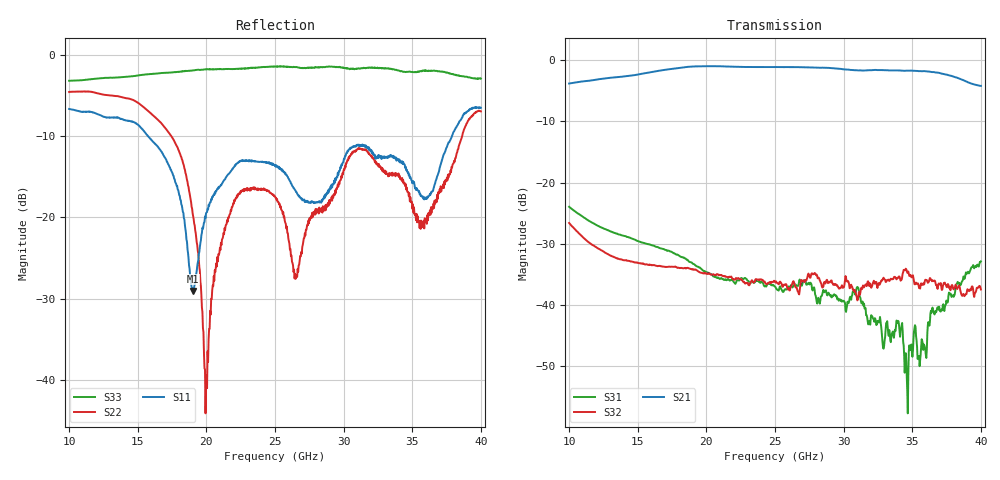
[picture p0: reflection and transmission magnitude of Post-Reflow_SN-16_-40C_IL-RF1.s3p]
!Agilent Technologies,N5245A,US49150155,A.09.90.19
!Agilent N5245A: A.09.90.19
!Date: Wednesday, November 14, 2018 00:00:33
!Correction: S11(Full 3 Port(1,2,3))
!S12(Full 3 Port(1,2,3))
!S13(Full 3 Port(1,2,3))
!S21(Full 3 Port(1,2,3))
!S22(Full 3 Port(1,2,3))
!S23(Full 3 Port(1,2,3))
!S31(Full 3 Port(1,2,3))
!S32(Full 3 Port(1,2,3))
!S33(Full 3 Port(1,2,3))
!S3P File: Measurements: <S11,S12,S13>,
!<S21,S22,S23>,
!<S31,S32,S33>:
# Hz S  dB  R 50
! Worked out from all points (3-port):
!   801 points, 10 GHz to 40 GHz, reference 50 ohm
!   strongest paths, dB at 10 GHz, 17.5 GHz, 25 GHz, 32.5 GHz, 40 GHz:
!     S21: -3.9, -1.5, -1.2, -1.7, -4.2
!     S32: -26.6, -33.7, -36.2, -36.7, -37.5
!     S31: -24.0, -31.4, -37.0, -42.8, -32.9
!   lowest |S11| = -29.0 dB at 19 GHz (marker M1), VSWR 1.07, Z = 46.6 - j0.352 ohm
!   |S11| at or under -10 dB: 15.73 GHz to 37.89 GHz (22.16 GHz wide, 82.7 % of centre)
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1e10  -6.68 -5.7  -3.85 -168.7  -23.97 57.8
      -3.85 -168.7  -4.60 -115.1  -26.61 -6.9
      -23.97 57.9  -26.60 -6.6  -3.22 49.7
1.4875e10  -8.48 -154.8  -2.44 80.3  -29.41 -30.9
           -2.44 80.3  -5.78 151.6  -33.02 -89.5
           -29.41 -30.6  -33.04 -89.4  -2.61 -55.6
1.9e10  -29.04 -173.9  -1.08 -17.5  -33.17 -112.3
        -1.07 -17.5  -19.50 73.3  -34.16 -179.9
        -33.21 -111.8  -34.13 -179.7  -1.94 -127.3
1.9975e10  -19.50 -133.8  -1.02 -41.5  -34.70 -126.8
           -1.02 -41.4  -40.57 139.5  -34.90 157.8
           -34.69 -126.9  -34.86 158.2  -1.83 -140.6
2.2e10  -13.83 -163.2  -1.11 -89.9  -36.30 -152.4
        -1.10 -89.9  -18.31 156.6  -35.80 109.7
        -36.25 -152.3  -35.79 109.6  -1.77 -169.5
2.5e10  -13.71 146.5  -1.16 -160.0  -37.01 157.2
        -1.16 -159.9  -17.45 86.3  -36.21 38.1
        -37.00 157.3  -36.18 38.4  -1.45 148.7
2.91625e10  -16.30 152.1  -1.33 99.3  -38.53 84.7
            -1.33 99.4  -17.94 -169.5  -36.37 -66.9
            -38.44 84.6  -36.40 -66.4  -1.48 89.3
3.31e10  -12.65 112.9  -1.68 4.2  -42.89 25.0
         -1.68 4.4  -14.37 67.4  -36.18 -147.6
         -42.94 26.2  -36.21 -147.6  -1.71 35.0
3.64375e10  -16.80 95.0  -1.99 -85.0  -40.73 25.3
            -1.98 -84.8  -18.75 -110.6  -36.09 106.5
            -40.77 24.6  -36.11 106.8  -1.99 -22.6
4e10  -6.53 70.4  -4.23 178.8  -32.84 -53.2
      -4.23 179.0  -6.98 93.1  -37.52 -73.5
      -32.87 -52.9  -37.45 -73.2  -2.96 -84.3
